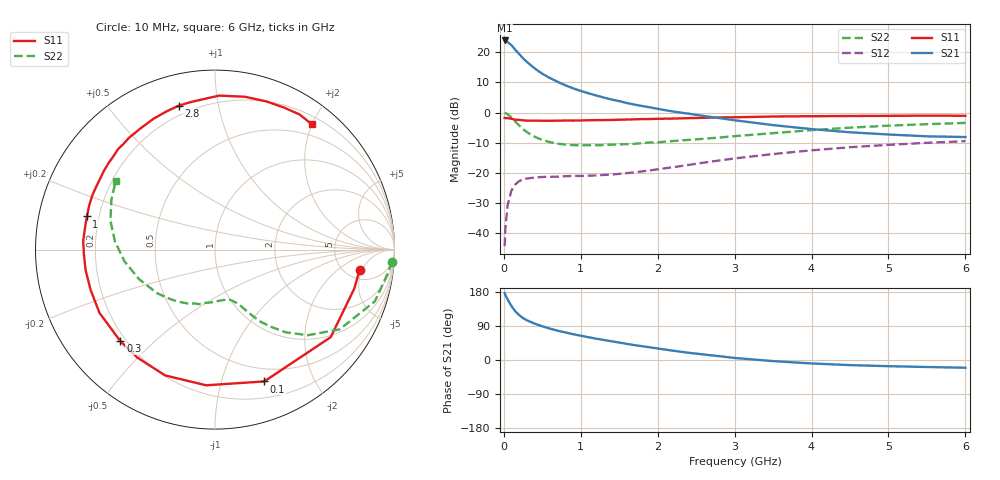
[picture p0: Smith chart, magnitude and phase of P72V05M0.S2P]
! SIEMENS Small Signal Semiconductors
! BFP196
! Si NPN RF Bipolar Junction Transistor in SOT143
! VCE = 2 V  IC = 5 mA
! Common Emitter S-Parameters:  May  1996
# GHz  S  MA  R  50
!  f  S11  S21  S12  S22
! GHz  MAG  ANG  MAG  ANG  MAG  ANG  MAG  ANG
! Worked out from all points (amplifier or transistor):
!   36 points, 10 MHz to 6 GHz, reference 50 ohm
!   highest |S21| = 24.0 dB at 10 MHz (marker M1)
!   |S21| within 3 dB of that: start of sweep to 145.8 MHz
!   unconditionally stable (mu >= 1): 1.118 GHz to 3.26 GHz; 5.766 GHz to end of sweep
!   at 250 MHz: K = 0.26, MSG = 20.2 dB, |S12| = -22.3 dB
!   at 1.4 GHz: K = 1.17, MAG = 10.0 dB, |S12| = -20.6 dB
!   at 6 GHz: K = 1.01, MAG = 0.0 dB, |S12| = -9.5 dB
!   S11 on the Smith chart (normalised r, x): 10 MHz: 6.74, -4.46; 100 MHz: 0.36, -1.38; 300 MHz: 0.18, -0.39; 1 GHz: 0.15, +0.12; 2.8 GHz: 0.15, +0.77; 6 GHz: 0.32, +2.00
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0.01  0.8136 -7.9  15.76 176.8  0.006 87.9  0.9872 -3.9
0.02  0.806 -15.6  15.43 171.2  0.012 81.9  0.9739 -7.4
0.05  0.8085 -37.1  14.8 159.4  0.0292 71.3  0.9364 -17.9
0.1  0.784 -69.5  13.09 142.0  0.0509 56.3  0.8246 -32.6
0.15  0.7577 -93.7  11 128.2  0.0641 45.2  0.7034 -42.7
0.2  0.754 -111.6  9.376 118.4  0.0725 37.7  0.6073 -49.4
0.25  0.741 -125.7  7.977 110.5  0.077 32.4  0.5283 -54.3
0.3  0.7337 -135.9  6.918 104.8  0.0798 29.2  0.4727 -57.9
0.4  0.7338 -151.3  5.421 96.0  0.0831 24.5  0.3955 -62.2
0.5  0.7285 -162.1  4.408 88.9  0.0848 21.8  0.3504 -65.0
0.6  0.7299 -171.0  3.733 82.8  0.0854 20.8  0.3222 -67.8
0.7  0.7311 -178.3  3.231 77.3  0.0859 20.7  0.3038 -70.7
0.8  0.7359 176.2  2.835 72.7  0.0873 20.7  0.2927 -73.2
1  0.7374 165.5  2.284 64.1  0.0882 22.3  0.2854 -78.2
1.1  0.7429 160.6  2.087 60.1  0.0891 23.7  0.2852 -81.3
1.6  0.7643 140.9  1.435 42.5  0.0983 31.5  0.2986 -97.3
2.2  0.7929 121.4  1.039 24.5  0.1234 38.3  0.3357 -116.4
2.8  0.8271 104.2  0.808 10.1  0.1592 38.6  0.3836 -136.7
3.5  0.8583 88.5  0.617 -2.9  0.2041 33.2  0.4541 -158.7
4.5  0.874 70.8  0.469 -13.5  0.2647 22.0  0.5598 175.2
5.5  0.8882 58.0  0.402 -18.5  0.3135 9.5  0.6399 154.5
6  0.8825 52.3  0.391 -20.4  0.3341 2.9  0.6719 145.5
